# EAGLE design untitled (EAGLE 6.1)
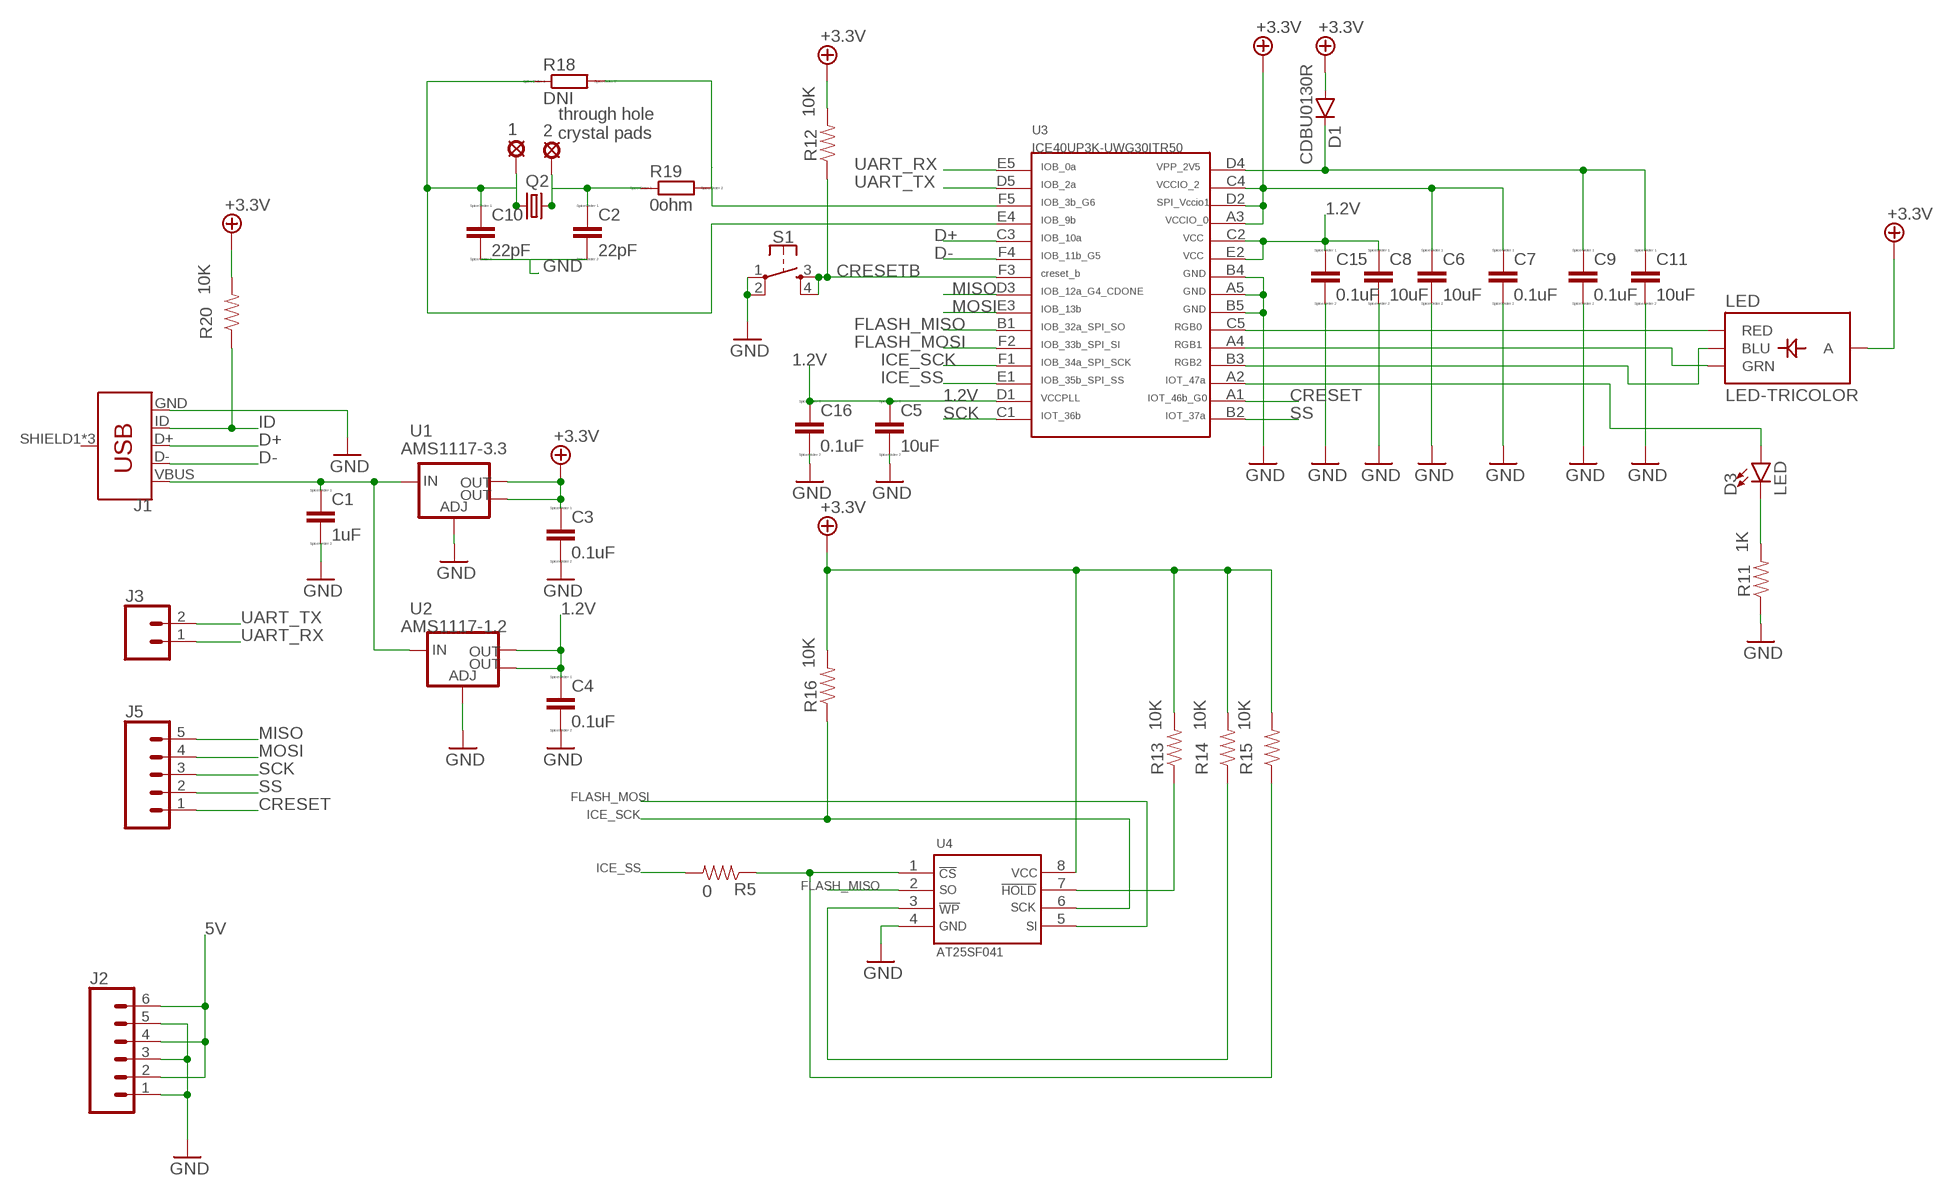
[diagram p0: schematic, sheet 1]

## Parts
1  LSP10  [LSP10]
2  LSP10  [LSP10]
C1  1uF  CC0402  [C0402]
C2  22pF  CC0402  [C0402]
C3  0.1uF  CC0402  [C0402]
C4  0.1uF  CC0402  [C0402]
C5  10uF  CC0402  [C0402]
C6  10uF  CC0402  [C0402]
C7  0.1uF  CC0402  [C0402]
C8  10uF  CC0402  [C0402]
C9  0.1uF  CC0402  [C0402]
C10  22pF  CC0402  [C0402]
C11  10uF  CC0402  [C0402]
C15  0.1uF  CC0402  [C0402]
C16  0.1uF  CC0402  [C0402]
D1  CDBU0130R  DIODE1  [SOD523]
D3  LED  LED0603  [LED-0603]
J1  USB_MICRO-B_FEMALE-SMT  [USB-B-MICRO-SMD]
J2  CONN_06NO_SILK_FEMALE_PTH  [1X06_NO_SILK]
J3  CONN_02  [1X02]
J5  CONN_05  [1X05]
LED  LED-TRICOLOR  [LED-TRICOLOR-SMD]
Q2  CRYSTALHC49UP  [HC49UP]
R5  0  RESISTOR0805-RES  [0805]
R11  1K  RESISTOR0603  [0603-RES]
R12  10K  RESISTOR0603  [0603-RES]
R13  10K  RESISTOR0603-RES  [0603-RES]
R14  10K  RESISTOR0603-RES  [0603-RES]
R15  10K  RESISTOR0603-RES  [0603-RES]
R16  10K  RESISTOR0603-RES  [0603-RES]
R18  DNI  RR0402  [R0402]
R19  0ohm  RR0402  [R0402]
R20  10K  RESISTOR0603  [0603-RES]
S1  MOMENTARY-SWITCH-SPST-2-SMD-4.6X2.8MM  [TACTILE_SWITCH_SMD_4.6X2.8MM]
U1  AMS1117-3.3  V_REG_LM1117SOT223  [SOT223]
U2  AMS1117-1.2  V_REG_LM1117SOT223  [SOT223]
U3  ICE40UP3K-UWG30ITR50  [WLSC-30]
U4  AT25SF041  [SO8]

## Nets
1.2V: C4.1 C5.1 C8.1 C15.1 C16.1 U2.2(OUT) U2.4(OUT) U3.C2 U3.D1 U3.E2
5: 1.MP C10.1 Q2.1 R18.1 U3.E4
5V: C1.1 J1.VBUS J2.2 J2.4 J2.6 U1.3(IN) U2.3(IN)
6: R18.2 R19.2 U3.F5
+3.3V: C3.1 C6.1 C7.1 D1.A LED.A R12.2 R13.2 R14.2 R15.2 R16.2 R20.2 U1.2(OUT) U1.4(OUT) U3.A3 U3.C4 U3.D2 U4.8
CRESET: J5.1 U3.A1
CRESETB: R12.1 S1.3 S1.4 U3.F3
D+: J1.D+ U3.C3
D-: J1.D- U3.F4
FLASH_MISO: U3.B1 U4.2
FLASH_MOSI: U3.F2 U4.5
GND: C1.2 C2.2 C3.2 C4.2 C5.2 C6.2 C7.2 C8.2 C9.2 C10.2 C11.2 C15.2 C16.2 J1.GND J2.1 J2.3 J2.5 R11.1 S1.1 S1.2 U1.1(ADJ) U2.1(ADJ) U3.A5 U3.B4 U3.B5 U4.4
ICE_SCK: R16.1 U3.F1 U4.6
ICE_SS: R5.2 U3.E1
ID: J1.ID R20.1
MISO: J5.5 U3.D3
MOSI: J5.4 U3.E3
N$4: R13.1 U4.7
N$6: R14.1 U4.3
N$7: R5.1 R15.1 U4.1
N$9: LED.R(RED) U3.C5
N$10: LED.G(GRN) U3.A4
N$11: LED.B(BLU) U3.B3
N$12: D3.A U3.A2
N$13: D3.C R11.2
N$18: C9.1 C11.1 D1.C U3.D4
N$24: 2.MP C2.1 Q2.2 R19.1
SCK: J5.3 U3.C1
SS: J5.2 U3.B2
UART_RX: J3.1 U3.E5
UART_TX: J3.2 U3.D5
Unconnected: J1.SHIELD1(SHIELD) J1.SHIELD2(SHIELD) J1.SHIELD3(SHIELD)

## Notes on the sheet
- through hole
   crystal pads

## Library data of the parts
1 2 = solpad:LSP10: SOLDER PAD
C1-C11 C15 C16 = eagle-ltspice:C: CAPACITOR, European symbol; SPICEMODEL: NONE; SPICEPREFIX: C
D1 = CDBU0130R:DIODE1
D3 = SparkFun-LED:LED: LED (Generic)
J1 = MICRO USB 105164-0001:USB_MICRO-B: USB Type Micro-B Connector Male/female and PTH/SMT variants SparkFun Products: SparkFun microB USB Breakout SparkFun USB microB Plug Breakout SparkFun ESP8266 Thing; PROD_ID: CONN-11752
J2 = SparkFun-Connectors:CONN_06: Multi connection point. Often used as Generic Header-pin footprint for 0.1 inch spaced/style header connections On any of the 0.1 inch spaced packages, you can populate with these: Break Away Headers - Straight (PRT-00116) Break Away Male Headers - Right Angle (PRT-00553) Female Headers (PRT-00115)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; PROD_ID: CONN-08437
J3 = SparkFun-Connectors:CONN_02: Multi connection point. Often used as Generic Header-pin footprint for 0.1 inch spaced/style header connections
J5 = SparkFun-Connectors:CONN_05: Multi connection point. Often used as Generic Header-pin footprint for 0.1 inch spaced/style header connections On any of the 0.1 inch spaced packages, you can populate with these: Break Away Headers - Straight (PRT-00116) Break Away Male Headers - Right Angle (PRT-00553) Female Headers (PRT-00115)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
LED = SparkFun-LED:LED-TRICOLOR: Tri-Color LED SMD Proven layout and schematic for triple color LED in SMD package - common anode. Spark Fun Electronics SKU : COM-07844
Q2 = crystal:CRYSTAL: CRYSTAL; OC_FARNELL: unknown; OC_NEWARK: unknown
R5 R11-R16 R20 = SparkFun-Resistors:RESISTOR: Resistor
R18 R19 = eagle-ltspice:R: RESISTOR, European symbol; SPICEMODEL: NONE; SPICEPREFIX: R
S1 = SparkFun-Switches:MOMENTARY-SWITCH-SPST-2: Momentary Switch (Pushbutton) - SPST - Two Circuits Normally-open (NO) SPST momentary switches (buttons, pushbuttons). Schematic symbol includes two switch circuits. Variants SMD-4.6MMX2.8MM - 4.60mm x 2.80mm Tactile Momentary Button Switch - Used on SparkFun SAMD21 Mini Breakout SMD-5.2MM - Mini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; PROD_ID: SWCH-13065
U1 U2 = SparkFun-IC-Power:V_REG_LM1117: Voltage Regulator LM1117 Standard adjustable voltage regulator but in SMD form. Spark Fun Electronics SKU : COM-00595; PROD_ID: VREG-08170
U3 = ICE40UP3K:ICE40UP3K-UWG30ITR50
U4 = AT25SF041:AT25SF041

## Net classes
0 default: width 0.15 mm, drill 0.305 mm

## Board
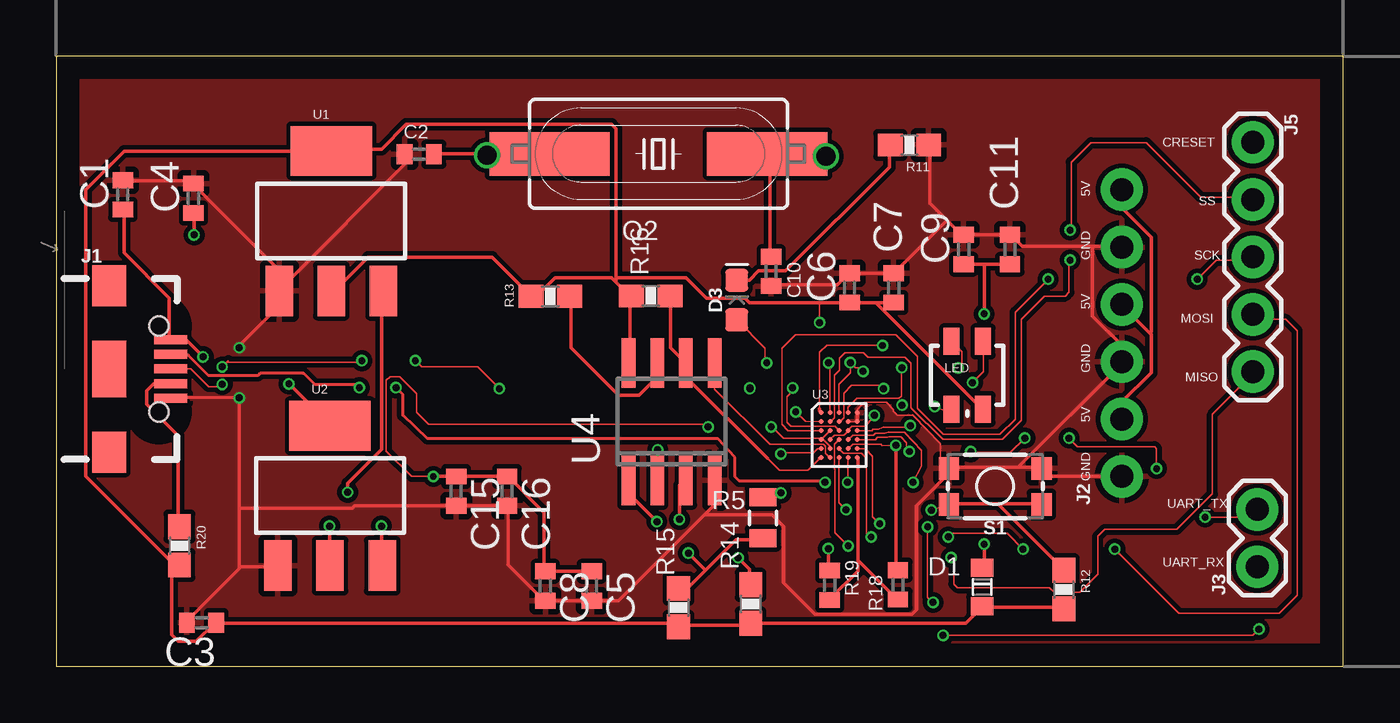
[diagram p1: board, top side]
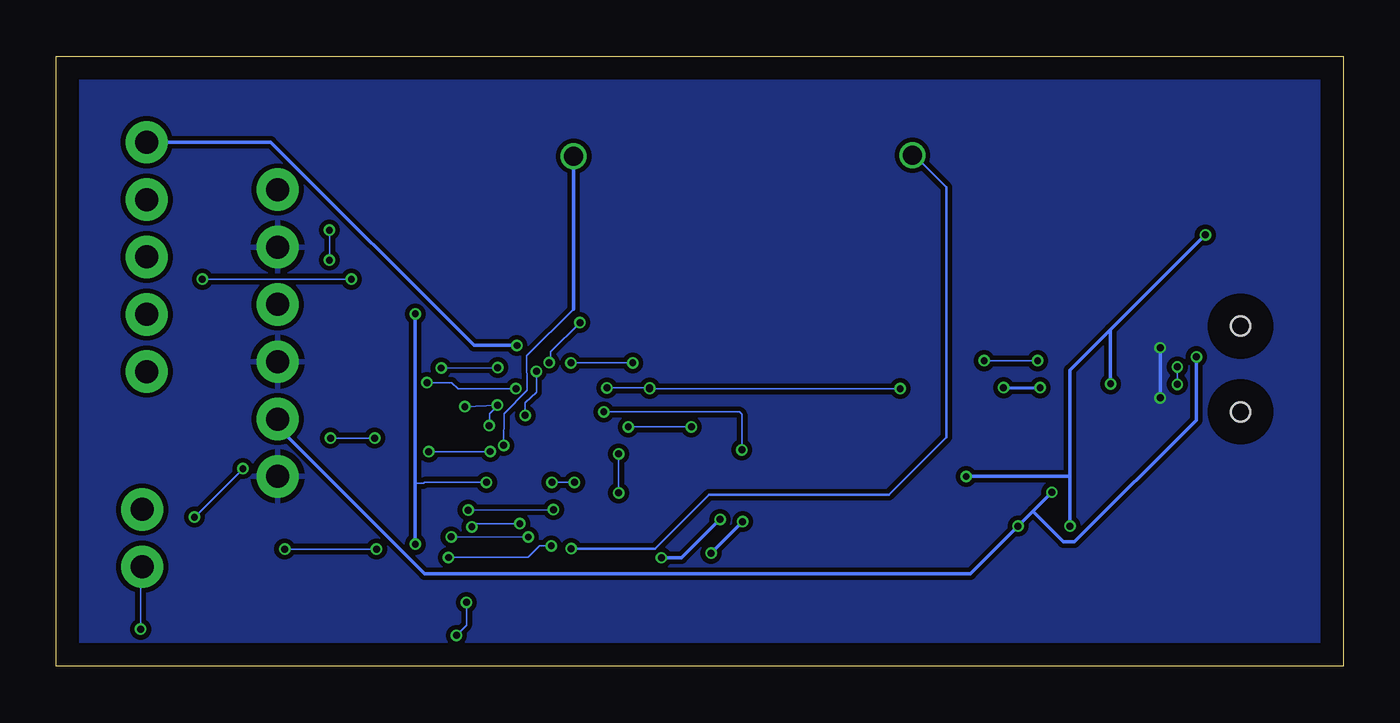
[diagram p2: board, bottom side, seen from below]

Size 57 x 27 mm. Coordinates in mm from the lower left corner, seen from the top.
Outline: 0,0 57,0 57,27 0,27 0,0
Copper layers (1*2*15*16): Top 0.035mm / dielectric 1.5mm / Route2 0.035mm / dielectric 0.15mm / Route15 0.035mm / dielectric 0.2mm / Bottom 0.035mm
Design rules: minimum track width 6mil, minimum drill 12mil, track to track 8mil, track to pad 8mil, pad to pad 8mil, via to via 8mil, smd to smd 8mil, copper to edge 40mil, drill to drill 8mil, minimum pad ring 5mil, minimum via ring 4mil, stop-mask expansion 4mil, vias tented up to drill 0mil, thermal gap 10mil

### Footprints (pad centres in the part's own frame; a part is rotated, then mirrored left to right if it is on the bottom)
LSP10 = drill 0.85: MP 0,0
C0402 = smd 0.7 x 0.9: 1 -0.65,0; 2 0.65,0
SOD523 = smd 0.8 x 1: A 1.1,0; C -0.6,0
LED-0603 = smd 1 x 1: A -0.877,0; C 0.877,0
USB-B-MICRO-SMD = smd 1.45 x 0.4: D+ 2.725,0; D- 2.725,0.65; GND 2.725,-1.3; ID 2.725,-0.65; VBUS 2.725,1.3 | smd 1.5 x 1.8: SHIELD1 0,3.685; SHIELD2 0,-3.685 | smd 1.5 x 2.5: SHIELD3 0,0 | hole 0.85: 2.2,1.9; 2.2,-1.9
1X06_NO_SILK = drill 1.016 pad 1.88: 1 0,0; 2 2.54,0; 3 5.08,0; 4 7.62,0; 5 10.16,0; 6 12.7,0
1X02 = drill 1.016 pad 1.88: 1 0,0; 2 2.54,0
1X05 = drill 1.016 pad 1.88: 1 0,0; 2 2.54,0; 3 5.08,0; 4 7.62,0; 5 10.16,0
LED-TRICOLOR-SMD = smd 0.7 x 1.2: A 0.7,-1.5; B 0.7,1.5; G -0.7,1.5; R -0.7,-1.5
HC49UP = smd 5.334 x 1.93: 1 -4.826,0; 2 4.826,0
0805 = smd 0.8 x 1.2: 1 -0.9,0; 2 0.9,0
0603-RES = smd 1.1 x 1: 1 -0.85,0; 2 0.85,0
R0402 = smd 0.7 x 0.9: 1 -0.65,0; 2 0.65,0
TACTILE_SWITCH_SMD_4.6X2.8MM = smd 0.9 x 1: 1 -2.05,-0.8; 2 2.05,-0.8; 3 2.05,0.8; 4 -2.05,0.8
SOT223 = smd 1.219 x 2.235: 1 -2.311,-3.099; 2 0,-3.099; 3 2.311,-3.099 | smd 3.6 x 2.2: 4 0,3.099
WLSC-30 = smd 0.22 x 0.22: A1 0,0; A2 0.4,0; A3 0.8,0; A4 1.2,0; A5 1.6,0; B1 0,-0.4; B2 0.4,-0.4; B3 0.8,-0.4; B4 1.2,-0.4; B5 1.6,-0.4; C1 0,-0.8; C2 0.4,-0.8; C3 0.8,-0.8; C4 1.2,-0.8; C5 1.6,-0.8; D1 0,-1.2; D2 0.4,-1.2; D3 0.8,-1.2; D4 1.2,-1.2; D5 1.6,-1.2; E1 0,-1.6; E2 0.4,-1.6; E3 0.8,-1.6; E4 1.2,-1.6; E5 1.6,-1.6; F1 0,-2; F2 0.4,-2; F3 0.8,-2; F4 1.2,-2; F5 1.6,-2
SO8 = smd 0.6 x 2.2: 1 -1.905,-2.6; 2 -0.635,-2.6; 3 0.635,-2.6; 4 1.905,-2.6; 5 1.905,2.6; 6 0.635,2.6; 7 -0.635,2.6; 8 -1.905,2.6

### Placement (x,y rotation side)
1  34.08,22.57 0 top
2  19.08,22.62 0 top
C1  2.94,20.87 90 top
C2  16.07,22.67 180 top
C3  6.43,1.92 180 top
C4  6.07,20.72 90 top
C5  23.71,3.55 270 top
C6  35.14,16.75 90 top
C7  37.09,16.75 90 top
C8  21.66,3.55 270 top
C9  40.19,18.45 90 top
C10  31.66,17.48 270 top
C11  42.24,18.45 90 top
C15  17.71,7.75 270 top
C16  19.96,7.75 270 top
D1  41.01,3.76 270 top
D3  30.14,16.21 90 top
J1  2.34,13.16 0 top
J2  47.2,8.4 90 top
J3  53.2,4.4 90 top
J5  53,23.2 270 top
LED  40.35,12.88 0 top
Q2  26.67,22.69 180 top
R5  31.3,6.57 90 top
R11  37.79,23.08 180 top
R12  44.63,3.39 270 top
R13  21.88,16.38 180 top
R14  30.75,2.75 270 top
R15  27.56,2.59 270 top
R16  26.33,16.4 180 top
R18  37.28,3.6 270 top
R19  34.26,3.58 270 top
R20  5.45,5.33 270 top
S1  41.59,7.96 180 top
U1  12.18,19.72 0 top
U2  12.12,7.55 0 top
U3  33.87,11.23 0 top
U4  27.25,10.83 0 top

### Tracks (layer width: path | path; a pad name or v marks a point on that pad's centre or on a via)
1.2V  (via drill 0.3)
  Top 0.076: U3.E2 34.3,9.66 34.3,9.72 33.95,10.07 U3.D1 | U3.D1 U3.C2 | U3.C2 34.28,10.46 34.27,10.44 U3.C2 | U3.D1 33.81,10.09 32.22,10.09 31.84,10.47 31.79,10.47 v31.67,10.59 | v28.87,10.59 28.75,10.71 16.5,10.71 15.97,11.24 15.97,12.06 15.21,12.82 14.78,12.82 14.62,12.65 14.62,9.53 15.74,8.4 v16.7,8.4
  Top 0.152: C5.1 C8.1 21.6,4.2 21.6,6.8 20,8.4 C16.1 C15.1 v16.7,8.4 | v6.1,19.1 6.1,20 C4.1 | v10.3,12.5 12.1,10.7 U2.4 | v12.1,6.2 12.1,4.5 U2.2
  Bottom 0.076: v31.67,10.59 v28.87,10.59
  Bottom 0.152: 10.3,14.9 v6.1,19.1 | v10.3,12.5 10.3,14.9 | 12.1,8.4 12.1,13.1 10.3,14.9 | 12.1,8.4 v12.1,6.2 | 12.1,8.4 v16.7,8.4
5  (via drill 0.3)
  Top 0.076: U3.E4 35.28,9.84 35.3,9.84 arc90 35.3,9.83 36.5,9.83 arc-90 36.56,9.76 v37.19,9.78
  Top 0.152: 31.6,22.5 31.6,18.2 C10.1 | 31.6,22.5 31.5,22.6 Q2.1 31.6,22.5 | v37.19,9.78 37.2,4.3 R18.1 | 31.6,22.5 34,22.5 1.MP
  Bottom 0.076: 34.1,15.8 36.16,13.73 36.15,12.21 37.17,11.18 v37.19,9.78 37.24,9.95 37.25,9.96 37.25,9.97
  Bottom 0.152: 34.1,15.8 34.1,22.5 1.MP
5V  (via drill 0.3)
  Top 0.152: J2.2 47.2,11.7 48.5,13 48.5,14.7 48.45,14.75 | 48.45,14.75 47.2,16 J2.4 | J2.6 47.2,20.3 48.5,19 48.5,14.8 48.45,14.75 | C1.1 3,20.2 3,18.3 5,16.3 5,14.5 J1.VBUS 5.1,14.4 5.8,14.4 v6.5,13.7 | v14.4,6.2 14.4,4.5 U2.3 | v12.9,7.7 12.9,8.1 14.4,9.6 14.4,16.6 U1.3
  Bottom 0.152: v12.9,7.7 13.75,6.85 | 13.75,6.85 v14.4,6.2 16.5,4.1 40.7,4.1 47.2,10.6 J2.2 | v6.5,13.7 6.5,10.9 11.9,5.5 12.4,5.5 13.75,6.85
6
  Top 0.152: 35.5,4.7 35.5,4.2 34.3,3 R19.2 | 35.5,4.7 35.5,9.2 U3.F5 | 35.5,4.7 37.2,3 R18.2
+3.3V  (via drill 0.3)
  Top 0.076: U3.D2 34.27,10.05 34.46,10.23 34.89,10.23 35.06,10.4 | 35.06,10.4 U3.C4 | U3.C4 35.07,10.41 35.06,10.4 | U3.A3 34.67,12.48 35.17,12.99 v35.17,13.44 35.15,13.46 35.41,13.21 35.58,13.21 v35.74,13.05 | v33.81,15.21 33.81,16.11 | 33.81,16.11 | 33.81,16.11 33.82,16.1 | U3.C4 35.07,10.45 35.25,10.62 35.84,10.62 v36.23,11.1
  Top 0.152: R12.2 44.6,2.6 41.1,2.6 D1.A 41,2.6 40.3,1.9 R14.2 30.7,1.9 30.6,1.8 27.6,1.8 R15.2 27.4,1.9 7.1,1.9 C3.1 7,1.9 6.2,1.1 5.4,1.1 5.1,1.4 5.1,4.1 5.4,4.4 R20.2 5.3,4.4 1.3,8.4 1.3,21.1 3,22.8 12.1,22.8 U1.4 12.2,22.9 14.4,22.9 15.5,24 24.6,24 24.8,23.8 24.8,17.2 | C7.1 36.3,16.1 | 36.3,16.1 C6.1 33.82,16.1 30.7,16.1 30.5,16.3 28.8,16.3 27.9,17.2 24.8,17.2 | 36.3,16.1 41,11.4 LED.A | 25.4,16.4 24.75,17.05 | 24.75,17.05 24.6,17.2 22.1,17.2 21.3,16.4 21.1,16.4 R13.2 21,16.4 19.3,18.1 13.8,18.1 12.4,16.7 12.2,16.7 U1.2 | 25.4,16.4 25.4,13.5 U4.8 | 25.4,16.4 R16.2 | 24.8,17.2 24.8,17.1 24.75,17.05
  Bottom 0.076: v35.17,13.44 35.1,13.51 35.1,13.92 v33.81,15.21 | v36.23,11.1 36.23,11.66 35.74,12.12 v35.74,13.05
CRESET  (via drill 0.3)
  Top 0.076: 33.8,11.4 33.8,13.89 34.12,14.22 36.58,14.22 v36.6,14.2
  Top 0.152: 33.8,11.4 33.8,11.3 U3.A1
  Bottom 0.152: v36.6,14.2 38.5,14.2 47.5,23.2 J5.1
CRESETB  (via drill 0.3)
  Top 0.076: U3.F3 34.67,7.24 v34.98,6.93 | v38.76,6.91 S1.3
  Top 0.152: 41.7,7.2 43.6,7.2 S1.4 | 41.7,7.2 39.6,7.2 S1.3 | 41.7,7.2 44.6,4.3 R12.1
  Bottom 0.076: v34.98,6.93 v38.76,6.91
D+  (via drill 0.3)
  Top 0.076: U3.C3 34.48,10.63 32.97,10.63 32.95,10.61 32.54,10.61 32.35,10.8 32.35,11.94 32.61,12.19 v32.61,12.32 | v30.72,12.32 v30.72,12.29 | v19.62,12.29 18.66,13.26 16.17,13.26 v15.9,13.53 | 7.62,13.53 v7.34,13.25 7.56,13.47 13.47,13.47 v13.53,13.53 | v7.34,12.48 7.25,12.38 6.74,12.38 5.94,13.18 5.08,13.18 J1.D+
  Bottom 0.076: v32.61,12.32 v30.72,12.32 | v30.72,12.29 v19.62,12.29 | v7.34,13.25 v7.34,12.48 | v15.9,13.53 v13.53,13.53
D-  (via drill 0.3)
  Top 0.076: U3.F4 35.07,8.22 v35.05,8.14 | v34.05,8.14 34,8.19
  Top 0.127: 34,8.19 30.26,8.19 30.06,8.39 30.06,9.25 29.3,10.07 16.44,10.07 15.35,11.1 15.35,12.02 v15.04,12.33 | v13.42,12.33 13.28,12.47 11.45,12.47 10.95,12.97 9.03,12.97 8.93,12.87 6.74,12.87 5.84,13.77 5.11,13.77 J1.D-
  Bottom 0.076: v35.05,8.14 v34.05,8.14
  Bottom 0.127: v15.04,12.33 v13.42,12.33
FLASH_MISO  (via drill 0.3)
  Top 0.076: U3.B1 33.18,10.84 v32.75,11.26 | v26.63,9.58 26.66,9.56 26.66,8.27 U4.2
  Bottom 0.076: v32.75,11.26 26.74,11.26 26.63,11.15 v26.63,9.58
FLASH_MOSI
  Top 0.076: U4.5 29.16,12.27 31.6,9.82 33.99,9.82 34.07,9.74 34.07,9.43 U3.F2
GND  (via drill 0.3)
  Top 0.076: U3.B4 U3.B5 | S1.2 39.16,9.17 39.17,9.86 37.94,11.12 37.93,11.13 37.91,11.12 37.26,11.12 37.09,11.29 37.09,11.36 36.77,11.68 35.79,11.68 35.63,11.52 35.48,11.37 35.48,11.11
  Top 0.127: 5.8,11.9 8.05,11.9 8.07,11.88 v8.1,11.88
  Top 0.152: U3.A5 35.5,11.2 35.48,11.11 U3.B5 | 42.6,8.8 39.6,8.8 S1.2 39.5,8.7 39.5,8.5 38.1,7.1 38.1,2.5 37.9,2.3 33.6,2.3 32.2,3.7 32.2,6.2 31.7,6.7 28.8,6.7 28.75,6.75 | 42.6,8.8 43.6,8.8 S1.1 44,8.4 J2.1 | 42.6,8.8 47.2,13.4 J2.3 47.2,14.2 45.9,15.5 45.9,18.6 | C10.2 31.7,16.9 34.6,16.9 35.1,17.4 C6.2 C7.2 39.45,19.75 | 39.45,19.75 40.1,19.1 C9.2 C11.2 42.3,19.1 42.8,18.6 45.9,18.6 | 39.45,19.75 38.7,20.5 38.7,23 R11.1 | 45.9,18.6 47.2,18.6 J2.5 | 28.75,6.75 24.9,2.9 C5.2 C8.2 21.6,2.9 20,4.5 20,7.1 C16.2 C15.2 13.2,7.1 13.1,7 8.1,7 | 28.75,6.75 29.1,7.1 29.1,8.2 U4.4 | 8.15,4.35 8.2,4.4 9.8,4.4 U2.1 | 8.15,4.35 5.8,2 C3.2 | C1.2 3,21.5 5.9,21.5 6,21.4 C4.2 6.1,21.3 10.3,17.1 | 10.3,17.1 9.9,16.7 U1.1 | 10.3,17.1 15.4,22.2 15.4,22.6 C2.2 | 5.8,11.9 5.1,11.9 J1.GND | U1.1 9.8,16.6 9.8,15.9 8.05,14.15 v8.1,14.1 | 10.3,17.1 U1.1 | v8.1,11.88 8.1,7 | 8.1,7 8.1,4.4 8.15,4.35
  Bottom 0.152: v8.1,14.1 v8.1,11.88
  pour Top (isolate 0.12): 0,27 57,27 57,0 0,0
  pour Bottom (isolate 0.12): 0,27 57,27 57,0 0,0
ICE_SCK
  Top 0.076: 33.8,9.2 33.8,9.18 33.3,8.68 32.03,8.68 31.5,9.21 31.5,9.2
  Top 0.152: 31.5,9.2 27.9,12.8 27.9,13.4 U4.6 27.8,13.5 27.2,14.1 27.2,16.4 R16.1 | 33.8,9.2 U3.F1
ICE_SS  (via drill 0.3)
  Top 0.076: U3.E1 33.73,9.63 33.53,9.44 32.14,9.44 v32.09,9.4 | v32.09,7.67 31.97,7.55 31.38,7.55 R5.2
  Bottom 0.076: v32.09,9.4 v32.09,7.67
ID
  Top 0.152: R20.1 5.4,6.2 5.4,10.2 4,11.6 4,12.2 4.3,12.5 5,12.5 J1.ID
MISO  (via drill 0.3)
  Top 0.076: U3.D3 34.47,9.83 34.47,8.73 34.48,8.71 34.48,5.92 v35.07,5.33 | v39.63,4.81 39.75,4.7 39.75,3.63 39.91,3.48 43.99,3.48 44.21,3.26 45.34,3.26 46.13,4.06 46.13,5.75 46.44,6.05 49.63,6.05 51.21,7.63 51.21,11.15 53.03,12.97 53.05,12.97 53.05,12.99 J5.5
  Bottom 0.076: v35.07,5.33 35.59,5.33 36.1,4.81 v39.63,4.81
MOSI  (via drill 0.3)
  Top 0.076: U3.E3 34.88,9.42 35.67,9.42 35.89,9.2 35.88,5.86 v36.09,5.72 | v39.51,5.72 39.66,5.87 42.13,5.87 v42.82,5.18 | v46.89,5.18 49.73,2.34 54.17,2.34 54.96,3.13 54.96,14.86 54.47,15.35 53.23,15.35 J5.4
  Bottom 0.076: v36.09,5.72 v39.51,5.72 | v42.82,5.18 v46.89,5.18
N$4
  Top 0.152: R13.1 22.8,16.3 22.8,14.1 24.9,12 25.8,12 26.6,12.8 26.6,13.4 U4.7
N$6  (via drill 0.3)
  Top 0.152: v30.2,4.8 30.7,4.3 30.7,3.6 R14.1 | v27.6,6.5 27.6,8 27.8,8.2 U4.3
  Bottom 0.152: v30.2,4.8 29.3,4.8 v27.6,6.5
N$7  (via drill 0.3)
  Top 0.152: 28.75,4.25 30.1,5.6 31.3,5.6 R5.1 | 28.75,4.25 28,3.5 27.6,3.5 R15.1 | v26.6,6.4 25.4,7.6 25.4,8.2 U4.1 | 28.75,4.25 v28,5
  Bottom 0.152: v28,5 v26.6,6.4
N$9  (via drill 0.3)
  Top 0.076: U3.C5 36.12,10.43 36.18,10.49 36.42,10.49 36.62,10.57 37.69,10.57 v37.83,10.65 | v38.91,11.49 39.26,11.34 39.66,11.34 39.66,11.37 LED.R
  Bottom 0.076: v38.91,11.49 v37.47,11.56 37.81,11.18 v37.83,10.65
N$10  (via drill 0.3)
  Top 0.076: U3.A4 35.07,11.46 35.47,11.86 37.33,11.86 37.42,11.96 37.42,13.09 v37.45,13.22 | v39.96,13.2 40.11,13.36 40.11,13.92 LED.G
  Bottom 0.076: v37.45,13.22 v39.96,13.2
N$11  (via drill 0.3)
  Top 0.076: U3.B3 34.72,10.83 34.88,10.99 34.88,12.09 35.23,12.44 36.49,12.44 v36.64,12.29 | v40.59,12.56 41.06,13.04 41.06,14.36 LED.B
  Bottom 0.076: v36.64,12.29 39.22,12.29 39.49,12.56 v40.59,12.56
N$12  (via drill 0.3)
  Top 0.076: U3.A2 34.27,13.37 v34.21,13.43 | v31.47,13.43 31.4,13.5 31.4,14.08 D3.A
  Bottom 0.076: v34.21,13.43 v31.47,13.43
N$13
  Top 0.152: D3.C 30.2,17.1 30.7,17.1 31.1,17.5 32.3,17.5 36.9,22.1 36.9,23 R11.2
N$18  (via drill 0.3)
  Top 0.076: U3.D4 35.28,10.23 36.19,10.23 36.28,10.31 36.7,10.31 36.83,10.37 37.57,10.37 38.33,9.56 38.33,8.84 v37.95,8.14
  Top 0.152: C11.1 41.1,17.8 | 41.1,17.8 C9.1 | v41.1,5.4 41.1,4.4 D1.C | 41.1,17.8 v41.1,15.6
  Bottom 0.076: v37.95,8.14 40.69,8.14 40.74,8.09 41.09,8.09 41.1,8.08
  Bottom 0.152: v41.1,15.6 41.1,8.08 v41.1,5.4
N$24  (via drill 0.3)
  Top 0.152: v34.2,5.2 34.2,4.3 R19.1 | C2.1 16.8,22.7 19,22.7 2.MP 19.1,22.7 21.8,22.7 Q2.2
  Bottom 0.103: v34.2,5.2 30.49,5.2 28.1,7.59 20.11,7.59 17.57,10.13 17.57,21.21 18.96,22.6 19.05,22.6 2.MP
  Bottom 0.152: 19.1,22.6 2.MP
SCK  (via drill 0.3)
  Top 0.076: U3.C1 32.41,10.43 32.14,10.71 32.14,14.08 32.73,14.68 37.19,14.68 38.14,13.73 38.14,11.41 39.29,10.26 41.8,10.26 42.47,10.94 42.47,15.68 v43.94,17.14 | v50.54,17.14 51.38,17.98 52.86,17.98 J5.3
  Bottom 0.076: v43.94,17.14 v50.54,17.14
SS  (via drill 0.3)
  Top 0.076: U3.B2 34.3,10.83 34.46,10.99 34.46,12.89 34.69,13.11 34.69,13.64 34.92,13.88 35.74,13.88 35.94,13.68 37.59,13.68 37.86,13.41 37.86,11.45 39.27,10.04 41.9,10.04 42.74,10.88 42.74,15.37 43.76,16.38 44.69,16.38 44.86,16.55 44.86,17.82 44.96,17.93 v44.91,17.98 | J5.2 52.89,20.77 50.7,20.77 48.28,23.19 45.83,23.19 44.96,22.32 44.96,19.36 v44.91,19.31
  Bottom 0.076: v44.91,19.31 v44.91,17.98
UART_RX  (via drill 0.3)
  Top 0.076: U3.E5 35.83,9.63 36.16,9.3 36.16,6.62 v36.47,6.31 | v38.6,6.17 38.6,3.06 v38.83,2.82 | v39.28,1.36 52.99,1.36 v53.27,1.63 | v53.27,4.31 53.24,4.34 53.24,4.36 J3.1
  Bottom 0.076: v36.47,6.31 38.46,6.31 v38.6,6.17 | v38.83,2.82 38.83,1.81 v39.28,1.36 | v53.27,1.63 v53.27,4.31
UART_TX  (via drill 0.3)
  Top 0.076: U3.D5 36.28,10.03 36.38,10.13 36.81,10.13 36.89,10.17 37.4,10.17 37.66,9.89 37.66,9.62 v37.78,9.5 | v40.51,9.49 40.54,9.47 42.27,9.47 v42.9,10.1 | v44.86,10.1 45.24,9.72 48.65,9.72 48.74,9.64 v48.74,8.74 | v50.88,6.6 52.81,6.6 53.2,6.98 J3.2
  Bottom 0.076: v37.78,9.5 v40.51,9.49 | v42.9,10.1 v44.86,10.1 | v48.74,8.74 v50.88,6.6

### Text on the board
tPlace: CRESET | 5V | SS | GND | SCK | 5V | MOSI | GND | MISO | 5V | GND | UART_TX | UART_RX

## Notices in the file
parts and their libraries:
SparkFun-IC-Power: Licensing: Creative Commons ShareAlike 4.0 International - https://creativecommons.org/licenses/by-sa/4.0
